(* Logix 5000 AddOnInstructionDefinition export B256_FRED; software revision 30.00 *)

ADD_ON_INSTRUCTION D_SHR   (* revision 1.0, vendor Ken Fischer, NSWCPD, C512 *)
// DINT bit shift right of the 32-bit argument Inp_A by Inp_B bits with paddding by zeros on the right
// Revision note:
// Rev1.0: TBD - Initial Release
VAR_IN_OUT
   Inp_A : DINT; {required}   // 64-bit Integer to be right circular rotated
END_VAR
VAR_INPUT
   Inp_B : INT; {required}   // Number of bits to shift
END_VAR
VAR_IN_OUT
   Out : DINT; {required}   // Result
END_VAR
VAR
   BSR_Cntrl : CONTROL := (LEN := 32);
   ONS : BOOL;
   Source_Bit : BOOL;
   Wrk_InpA : DINT[2];
END_VAR

ROUTINE Logic   (* ladder *)
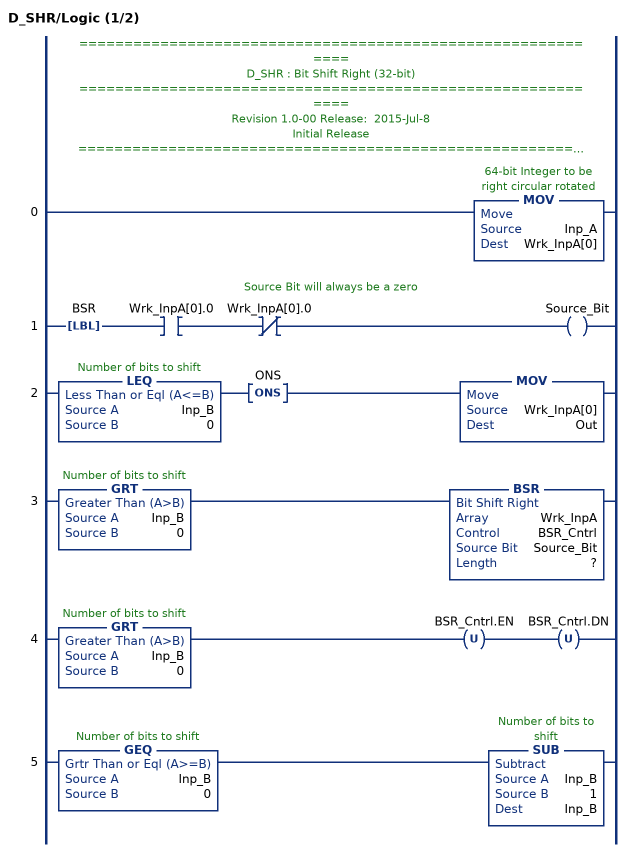
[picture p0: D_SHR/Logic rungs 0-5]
   // ============================================================
   // D_SHR : Bit Shift Right (32-bit)
   // ============================================================
   // Revision 1.0-00 Release:  2015-Jul-8
   // Initial Release
   // ============================================================
   // Performs a right bit shift of the 32-bit argument Inp_A by the
   // number of bits defined in the 16-bit argument Inp_B, with padding by zeros.
   0: MOV(Inp_A,Wrk_InpA[0]);
   // Source Bit will always be a zero
   1: LBL(BSR)XIC(Wrk_InpA[0].0)XIO(Wrk_InpA[0].0)OTE(Source_Bit);
   2: LEQ(Inp_B,0)ONS(ONS)MOV(Wrk_InpA[0],Out);
   3: GRT(Inp_B,0)BSR(Wrk_InpA,BSR_Cntrl,Source_Bit,?);
   4: GRT(Inp_B,0)OTU(BSR_Cntrl.EN)OTU(BSR_Cntrl.DN);
   5: GEQ(Inp_B,0)SUB(Inp_B,1,Inp_B);
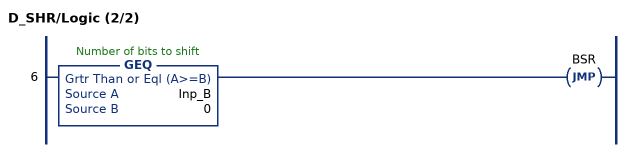
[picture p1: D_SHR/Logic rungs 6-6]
   6: GEQ(Inp_B,0)JMP(BSR);
END_ROUTINE
END_ADD_ON_INSTRUCTION

ADD_ON_INSTRUCTION B256_FRED   (* revision 1.0 20170916, vendor Kenneth A. Fischer *)
// fast_reduce:  reduce by propagating the carries starting at a particular offset and stoping once the carry becomes zero
// Revision note:
// Rev1.0: 20170916 - Initial Release
VAR_IN_OUT
   Inp_C : DINT[22]; {required}
END_VAR
VAR_INPUT
   Inp_offset : INT; {required}
END_VAR
VAR
   i : INT;
   carry : DINT;
   D_SHR : D_SHR;
END_VAR

ROUTINE Logic   (* ladder *)
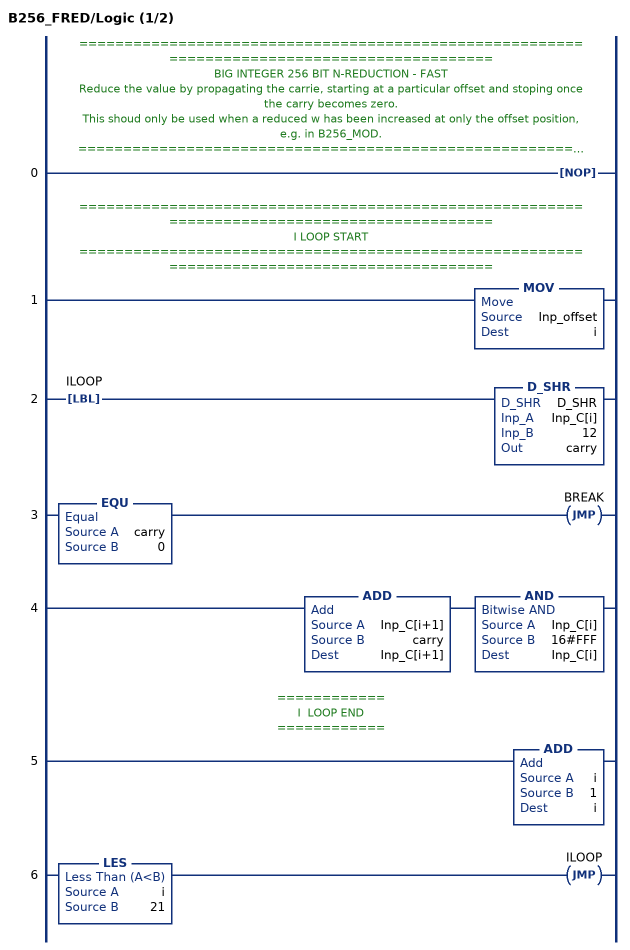
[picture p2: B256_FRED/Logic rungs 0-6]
   // ============================================================================================
   // BIG INTEGER 256 BIT N-REDUCTION - FAST
   // Reduce the value by propagating the carrie, starting at a particular offset and stoping once the carry becomes zero.
   // This shoud only be used when a reduced w has been increased at only the offset position, e.g. in B256_MOD.
   // ============================================================================================
   0: NOP();
   // ============================================================================================
   // I LOOP START
   // ============================================================================================
   1: MOV(Inp_offset,i);
   2: LBL(ILOOP)D_SHR(D_SHR,Inp_C[i],12,carry);
   3: EQU(carry,0)JMP(BREAK);
   4: ADD(Inp_C[i+1],carry,Inp_C[i+1])AND(Inp_C[i],16#FFF,Inp_C[i]);
   // ============
   // I  LOOP END
   // ============
   5: ADD(i,1,i);
   6: LES(i,21)JMP(ILOOP);
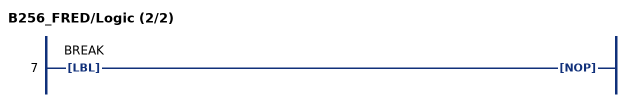
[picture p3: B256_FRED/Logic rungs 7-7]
   7: LBL(BREAK)NOP();
END_ROUTINE
END_ADD_ON_INSTRUCTION
